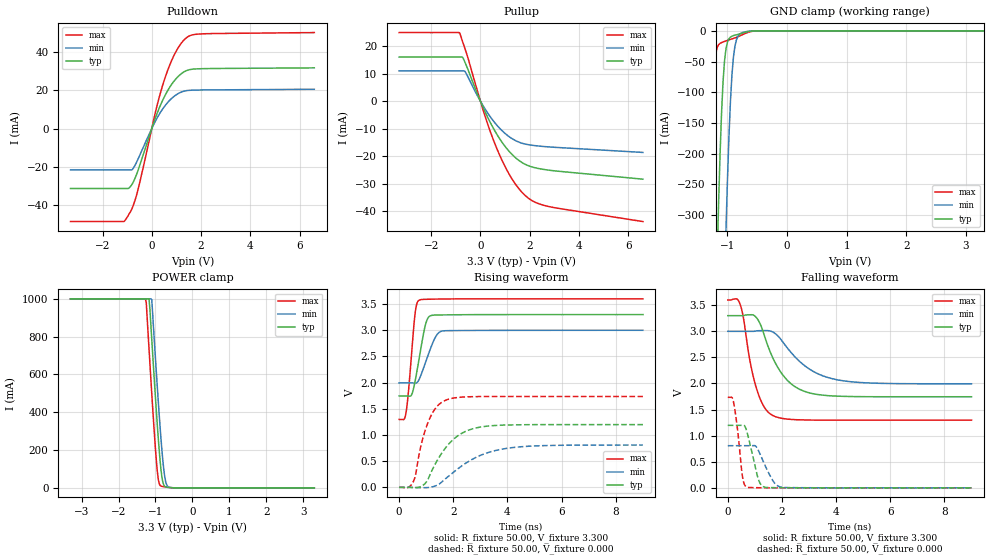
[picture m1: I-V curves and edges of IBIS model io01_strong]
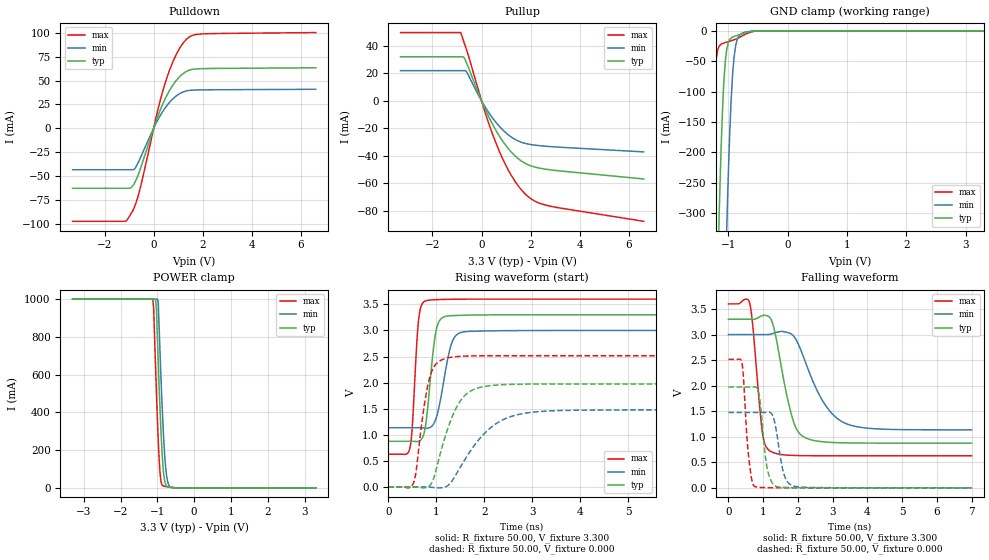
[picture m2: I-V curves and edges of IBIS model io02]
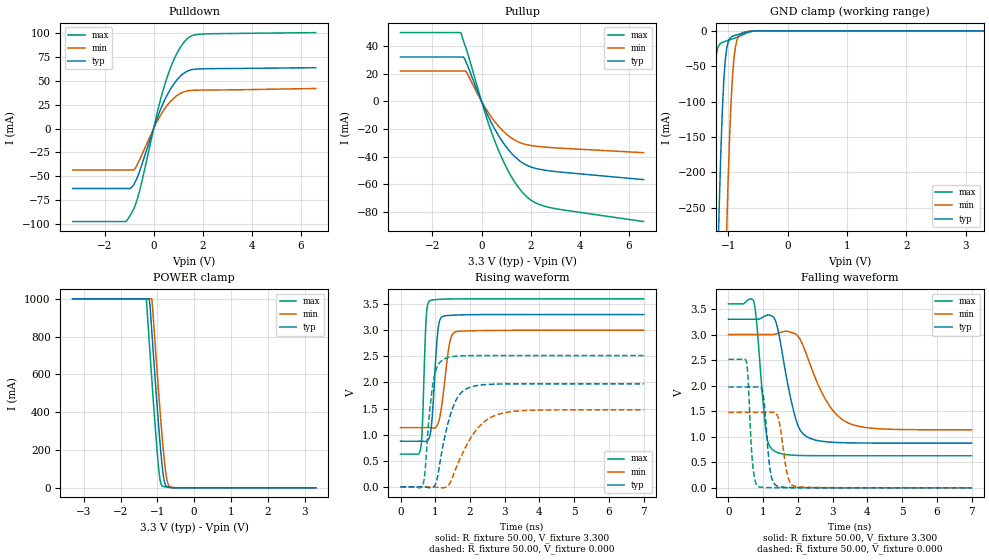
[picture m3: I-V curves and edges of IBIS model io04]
[IBIS Ver]   3.2
[File name]   rx630_177tflga.ibs
[File Rev]   2.00
[Date]   Sep 10, 2012
[Source]   From silicon level SPICE model at
   Renesas Electronics Corporation
[Notes]
|   Renesas Microcomputer RX630 Group
|   RX630 177pin TFLGA
|   VCCQ : 3.30V
|(1) This IBIS file checked the format with ibischk5.
|   Format Error and Warning are 0.
|(2) Temperature described Tj.
|   Tj[deg]
|   Typical   45.0
|   Minimum   105.0
|   Maximum   -40.0
|(3) History
|   Rev 1.00  2012.3.22
|   New creation by Hitachi ULSI Systems Co,.Ltd.
|   Rev 2.00  2012.09.10
|   Some IO Models were changed
|   by Renesas Electronics Corporation
[Disclaimer]
   This information is for modeling purposes only,
   and is not guaranteed.
[Copyright]   Copyright 2012, Renesas Electronics Corporation ,
   All Rights Reserved
[Component]   rx630_177tflga
[Manufacturer]  Renesas Electronics Corporation
[Package]
|   typ   min   max
R_pkg   358m   358m   358m
L_pkg   1.7nH   1.7nH   1.7nH
C_pkg   0.26pF   0.26pF   0.26pF
[Pin] signal_name   model_name
A1   AVSS0   GND
A2   AVCC0   POWER
A3   VREFL0   GND
A4   P42   io14
A5   P46   io14
A6   VCC   POWER
A7   VSS   GND
A8   P94   io07
A9   PK0   io04
A10   P97   io07
A11   PD6   io01
A12   P60   io07
A13   P63   io07
A14   PE1   io01
A15   PE2   io01
B1   P05   io02
B2   P07   io06
B3   P40   io14
B4   P41   io14
B5   P47   io14
B6   P91   io01
B7   P92   io01
B8   PD1   io01
B9   P96   io07
B10   PD4   io01
B11   PG1   io07
B12   PK3   io04
B13   P64   io07
B14   PE0   io01
B15   PE3   io01
C1   VREFL   GND
C2   VREFH   POWER
C3   VREFH0   POWER
C4   P43   io14
C5   P45   io14
C6   P90   io01
C7   PD0   io01
C8   PD2   io01
C9   PD3   io01
C10   PG0   io07
C11   PK2   io04
C12   P62   io07
C13   PE4   io01
C14   PK4   io04
C15   P70   io07
D1   P01   io01
D2   P02   io01
D3   P03   io02
D4   P00   io01
D5   P44   io14
D6   P93   io01
D7   P95   io07
D8   PK1   io04
D9   PD5   io01
D10   PD7   io01
D11   P61   io07
D12   PE5   io01
D13   PK5   io04
D14   PE7   io01
D15   P65   io07
E1   PJ5   io04
E2   EMLE   input06
E3   PF5   io04
E4   VSS   GND
E5   NC   NC
E12   PE6   io01
E13   PG2   io07
E14   PG3   io07
E15   P67   io08
F1   VBATT   POWER
F2   VCL   POWER
F3   PJ3   io04
F4   BSCANP   input03
F12   P66   io07
F13   PG4   io07
F14   PA0   io07
F15   VSS   GND
G1   XCIN   NC
G2   XCOUT   NC
G3   MD   io04
G4   PF4   io04
G12   PG5   io04
G13   PG6   io07
G14   PA1   io08
G15   VCC   POWER
H1   P37   io05
H2   VSS   GND
H3   RES#   input02
H4   P35   input01
H12   PA4   io08
H13   PA3   io08
H14   PA2   io08
H15   PG7   io07
J1   P36   io03
J2   VCC   POWER
J3   P34   io06
J4   PF3   io04
J12   PA5   io07
J13   PK6   io04
J14   PA7   io07
J15   PA6   io08
K1   P33   io06
K2   P32   io21
K3   PF2   io04
K4   PF1   io04
K12   PB2   io08
K13   P71   io07
K14   PK7   io04
K15   PB0   io08
L1   P31   io21
L2   P30   io21
L3   PF0   io04
L4   P25   io06
L12   PB6   io08
L13   PB3   io08
L14   PB1   io08
L15   P72   io07
M1   P27   io07
M2   P26   io07
M3   P24   io06
M4   P86   io04
M5   P13   io18
M6   P56   io08
M7   P54   io08
M8   P53   io04
M9   P50   io08
M10   PC5   io08
M11   P81   io06
M12   P77   io08
M13   PB7   io08
M14   PB5   io08
M15   PB4   io08
N1   PH5   io04
N2   P23   io06
N3   P22   io06
N4   P15   io06
N5   P12   io18
N6   P57   io08
N7   P55   io08
N8   PL2   io04
N9   P51   io08
N10   PC7   io08
N11   P82   io06
N12   PC3   io08
N13   PC0   io17
N14   P73   io07
N15   PL0   io04
P1   PH4   io04
P2   P17   io15
P3   P87   io04
P4   P14   io06
P5   P10   io04
P6   VCC_USB   POWER
P7   VSS_USB   GND
P8   PL3   io04
P9   P52   io08
P10   P83   io04
P11   PC6   io08
P12   PC4   io08
P13   PC2   io08
P14   P75   io08
P15   PL1   io04
R1   P21   io16
R2   P20   io16
R3   P16   io15
R4   P85   io04
R5   P11   io04
R6   USB0_DM   io09
R7   USB0_DP   io09
R8   PL4   io04
R9   P84   io04
R10   VSS   GND
R11   VCC   POWER
R12   P80   io06
R13   P76   io08
R14   P74   io08
R15   PC1   io17
[Diff Pin]   inv_pin   vdiff   tdelay_typ   tdelay_min   tdelay_max
R6   R7   0.000V   0.000s   NA   NA
[Model Selector]   io01
io01_strong   driver strength strong
io01_weak   driver strength weak
[Model Selector]   io07
io07_strong   driver strength strong
io07_weak   driver strength weak
[Model Selector]   io08
io08_strong   driver strength strong
io08_weak   driver strength weak
[Model Selector]   io15
io15a   driver strength strong
io15b   I2C buffer 1
[Model Selector]   io16
io16a   driver strength strong
io16b   I2C buffer 2
[Model Selector]   io17
io17a_strong   driver strength strong
io17a_weak   driver strength weak
io17b   I2C buffer 3
[Model Selector]   io18
io18a   driver strength strong
io18b   I2C buffer 4
| Models and submodels in the file (27): io01_strong (I/O), io01_weak (I/O), io02 (I/O), io03 (I/O), io04 (I/O), io05 (I/O), io06 (I/O), io07_strong (I/O), io07_weak (I/O), io08_strong (I/O), io08_weak (I/O), io09 (I/O), io14 (I/O), io15a (I/O), io15b (I/O_open_drain), io16a (I/O), io16b (I/O_open_drain), io17a_strong (I/O), io17a_weak (I/O), io17b (I/O_open_drain), io18a (I/O), io18b (I/O_open_drain), io21 (I/O), input01 (Input), input02 (Input), input03 (Input), input06 (Input)
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[Model]   io01_strong
Model_type   I/O
Polarity   Non-Inverting
Enable   Active-High
Vinl  =   0.660V
Vinh  =   2.640V
Vmeas =   1.650V
Cref  =   30.00pF
| variable   typ   min   max
C_comp   5.910pF   5.910pF   5.910pF
| variable   typ   min   max
[Temperature Range]   45.000   105.000   -40.000
| variable   typ   min   max
[Voltage Range]   3.300V   3.000V   3.600V
| variable   typ   min   max
[Pullup Reference]   3.300V   3.000V   3.600V
| variable   typ   min   max
[Pulldown Reference]   0.000V   0.000V   0.000V
| variable   typ   min   max
[POWER Clamp Reference] 3.300V   3.000V   3.600V
| variable   typ   min   max
[GND Clamp Reference]   0.000V   0.000V   0.000V
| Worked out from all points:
|   slope of the pulldown table from 0 to 0.495 V, typ, clamps not added: 30.7 ohm
|   slope of the pullup table from 0 to 0.495 V, typ, clamps not added: 52.9 ohm
|   GND clamp passes 1 mA (typ) near -0.63 V on its own axis
|   POWER clamp passes 1 mA (typ) near -0.58 V on its own axis
|   rising waveform, R_fixture 50.00, V_fixture 3.300: 20-80 % time 321ps typ, 432ps min, 222ps max; typ from 1.75 V to 3.3 V
|   rising waveform, R_fixture 50.00, V_fixture 0.000: 20-80 % time 961ps typ, 1.48ns min, 553ps max; typ from 0 V to 1.2 V
|   falling waveform, R_fixture 50.00, V_fixture 3.300: 20-80 % time 902ps typ, 1.27ns min, 542ps max; typ from 3.3 V to 1.75 V
|   falling waveform, R_fixture 50.00, V_fixture 0.000: 20-80 % time 324ps typ, 446ps min, 218ps max; typ from 1.2 V to 0 V
[Pulldown]
| io01_strong Pulldown rx630
| Thu Mar 22 17:15:49 2012
| voltage   I(typ)   I(min)   I(max)
-3.3V     -31.31mA   -21.63mA   -48.57mA
-1.15V    -31.31mA   -21.63mA   -48.57mA
-1.025V   -31.31mA   -21.63mA   -46.81mA
-800mV    -29.1mA    -21.49mA   -41.71mA
-600mV    -23.34mA   -17.13mA   -33.95mA
175mV     6.49mA     4.538mA    9.911mA
525mV     16.92mA    11.68mA    25.93mA
950mV     25.49mA    17.23mA    39.38mA
1.4V      30.18mA    19.75mA    47.31mA
1.7V      31.04mA    20.05mA    49.02mA
2.1V      31.26mA    20.14mA    49.45mA
6.6V      31.67mA    20.5mA     50.09mA
[Pullup]
| io01_strong Pullup rx630
| Thu Mar 22 17:15:49 2012
| voltage   I(typ)   I(min)   I(max)
-3.3V     16.04mA    10.98mA    24.94mA
-850mV    16.04mA    10.98mA    24.94mA
-725mV    15.94mA    10.98mA    21.66mA
-625mV    14.1mA     10.75mA    19.05mA
175mV     -3.59mA    -2.649mA   -5.083mA
700mV     -12.53mA   -9.072mA   -17.96mA
1V        -16.45mA   -11.75mA   -23.79mA
1.325V    -19.76mA   -13.87mA   -28.89mA
1.95V     -23.51mA   -15.85mA   -35.33mA
2.3V      -24.41mA   -16.28mA   -37.1mA
2.9V      -25.25mA   -16.74mA   -38.59mA
6.6V      -28.4mA    -18.67mA   -43.82mA
[GND Clamp]
| io01_strong GNDClamp rx630
| Thu Mar 22 17:15:49 2012
| voltage   I(typ)   I(min)   I(max)
-3.3V     -1A        -1A        -1A
-1.325V   -1A        -1A        -369.2mA
-1.3V     -928.6mA   -1A        -269.7mA
-1.25V    -694.8mA   -1A        -112.6mA
-1.175V   -376mA     -953.3mA   -27.44mA
-1.15V    -283.8mA   -837.7mA   -22.69mA
-1.075V   -83.42mA   -512.2mA   -18.16mA
-1.025V   -28.94mA   -323mA     -16.39mA
-925mV    -8.707mA   -71.38mA   -13.1mA
-850mV    -6.468mA   -14.65mA   -10.64mA
-675mV    -1.81mA    -1.082mA   -3.186mA
3.3V      0A         0A         0A
[POWER Clamp]
| io01_strong PWRClamp rx630
| Thu Mar 22 17:15:49 2012
| voltage   I(typ)   I(min)   I(max)
-3.3V     1A         1A         1A
-1.275V   1A         1A         1A
-1.25V    1A         1A         982.1mA
-1.175V   1A         1A         736.6mA
-1.1V     784.3mA    995.9mA    498mA
-1V       476.2mA    683.1mA    204.7mA
-950mV    332.1mA    533mA      87.52mA
-875mV    143.3mA    321.7mA    12.76mA
-825mV    55.42mA    197.2mA    7.873mA
-750mV    8.12mA     59.94mA    5.513mA
-625mV    1.619mA    2.607mA    2.132mA
3.3V      0A         0A         0A
[Ramp]
dV/dt_r   0.719/960.74p  0.485/1.48n   1.041/552.35p
dV/dt_f   0.933/901.13p  0.604/1.27n   1.382/541.71p
R_load = 50.00ohm
[Rising Waveform]
| io01_strong Rising-High rx630
| Thu Mar 22 17:15:49 2012
R_fixture = 50.00
V_fixture = 3.300
V_fixture_min = 3.000
V_fixture_max = 3.600
C_fixture = 0.00pF
| Time   V(typ)   V(min)   V(max)
0s        1.746V     1.994V     1.297V
250ps     1.746V     1.994V     1.413V
450ps     1.759V     1.994V     2.489V
580ps     2.004V     1.989V     3.28V
645ps     2.183V     1.996V     3.491V
740ps     2.465V     2.064V     3.575V
1.045ns   3.216V     2.49V      3.592V
1.35ns    3.291V     2.878V     3.596V
1.585ns   3.293V     2.985V     3.598V
9ns       3.3V       3V         3.6V
[Rising Waveform]
| io01_strong Rising-Low rx630
| Thu Mar 22 17:15:49 2012
R_fixture = 50.00
V_fixture = 0.000
C_fixture = 0.00pF
| Time   V(typ)   V(min)   V(max)
0s        0V         0V         0V
510ps     -7mV       0V         95mV
605ps     -9mV       -1mV       236mV
840ps     25mV       -7mV       868mV
1.075ns   164mV      -4mV       1.25V
1.385ns   494mV      37mV       1.537V
1.755ns   781mV      183mV      1.672V
2.55ns    1.09V      490mV      1.729V
3.975ns   1.191V     745mV      1.735V
9ns       1.198V     808mV      1.735V
[Falling Waveform]
| io01_strong Falling-High rx630
| Thu Mar 22 17:15:49 2012
R_fixture = 50.00
V_fixture = 3.300
V_fixture_min = 3.000
V_fixture_max = 3.600
C_fixture = 0.00pF
| Time   V(typ)   V(min)   V(max)
0s        3.3V       3V         3.6V
445ps     3.3V       3V         3.533V
575ps     3.301V     3V         3.268V
825ps     3.317V     3V         2.418V
1.03ns    3.279V     3.006V     1.959V
1.325ns   2.961V     3.013V     1.567V
1.65ns    2.506V     2.99V      1.39V
2.46ns    1.947V     2.523V     1.308V
3.835ns   1.763V     2.095V     1.297V
9ns       1.746V     1.994V     1.297V
[Falling Waveform]
| io01_strong Falling-Low rx630
| Thu Mar 22 17:15:49 2012
R_fixture = 50.00
V_fixture = 0.000
C_fixture = 0.00pF
| Time   V(typ)   V(min)   V(max)
0s        1.198V     808mV      1.735V
210ps     1.198V     808mV      1.65V
350ps     1.198V     808mV      1.163V
545ps     1.199V     808mV      210mV
710ps     1.068V     808mV      13mV
1.12ns    182mV      727mV      3mV
1.35ns    15mV       460mV      1mV
1.71ns    4mV        104mV      1mV
2.015ns   2mV        10mV       0V
9ns       0V         0V         0V
[Model]   io02
Model_type   I/O
Polarity   Non-Inverting
Enable   Active-High
Vinl  =   0.660V
Vinh  =   2.640V
Vmeas =   1.650V
Cref  =   30.00pF
| variable   typ   min   max
C_comp   4.810pF   4.810pF   4.810pF
| variable   typ   min   max
[Temperature Range]   45.000   105.000   -40.000
| variable   typ   min   max
[Voltage Range]   3.300V   3.000V   3.600V
| variable   typ   min   max
[Pullup Reference]   3.300V   3.000V   3.600V
| variable   typ   min   max
[Pulldown Reference]   0.000V   0.000V   0.000V
| variable   typ   min   max
[POWER Clamp Reference] 3.300V   3.000V   3.600V
| variable   typ   min   max
[GND Clamp Reference]   0.000V   0.000V   0.000V
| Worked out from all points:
|   slope of the pulldown table from 0 to 0.495 V, typ, clamps not added: 15.3 ohm
|   slope of the pullup table from 0 to 0.495 V, typ, clamps not added: 26.5 ohm
|   GND clamp passes 1 mA (typ) near -0.60 V on its own axis
|   POWER clamp passes 1 mA (typ) near -0.56 V on its own axis
|   rising waveform, R_fixture 50.00, V_fixture 3.300: 20-80 % time 160ps typ, 229ps min, 107ps max; typ from 0.875 V to 3.3 V
|   rising waveform, R_fixture 50.00, V_fixture 0.000: 20-80 % time 439ps typ, 750ps min, 233ps max; typ from 0 V to 1.97 V
|   falling waveform, R_fixture 50.00, V_fixture 3.300: 20-80 % time 438ps typ, 788ps min, 230ps max; typ from 3.3 V to 0.875 V
|   falling waveform, R_fixture 50.00, V_fixture 0.000: 20-80 % time 184ps typ, 224ps min, 154ps max; typ from 1.97 V to 0 V
[Pulldown]
| io02_strong Pulldown rx630
| Thu Mar 22 17:15:49 2012
| voltage   I(typ)   I(min)   I(max)
-3.3V     -62.65mA   -43.27mA   -97.17mA
-1.15V    -62.65mA   -43.27mA   -97.17mA
-1.025V   -62.65mA   -43.27mA   -93.54mA
-800mV    -58.14mA   -42.96mA   -83.35mA
-600mV    -46.61mA   -34.21mA   -67.78mA
175mV     12.96mA    9.063mA    19.79mA
550mV     35.03mA    24.16mA    53.7mA
950mV     50.92mA    34.42mA    78.67mA
1.4V      60.32mA    39.47mA    94.54mA
1.7V      62.04mA    40.07mA    97.97mA
2.1V      62.48mA    40.25mA    98.84mA
6.6V      63.3mA     40.84mA    100.1mA
[Pullup]
| io02_strong Pullup rx630
| Thu Mar 22 17:15:49 2012
| voltage   I(typ)   I(min)   I(max)
-3.3V     32.07mA    21.98mA    49.71mA
-850mV    32.07mA    21.98mA    49.71mA
-725mV    31.79mA    21.98mA    43.1mA
-625mV    28.07mA    21.44mA    37.9mA
150mV     -6.167mA   -4.559mA   -8.713mA
675mV     -24.26mA   -17.6mA    -34.7mA
975mV     -32.23mA   -23.07mA   -46.52mA
1.3V      -39mA      -27.43mA   -56.92mA
1.925V    -46.81mA   -31.61mA   -70.21mA
2.3V      -48.81mA   -32.55mA   -74.14mA
2.8V      -50.28mA   -33.35mA   -76.77mA
6.6V      -56.92mA   -37.21mA   -87.76mA
[GND Clamp]
| io02_strong GNDClamp rx630
| Thu Mar 22 17:15:49 2012
| voltage   I(typ)   I(min)   I(max)
-3.3V     -1A        -1A        -1A
-1.325V   -1A        -1A        -406.6mA
-1.3V     -983.2mA   -1A        -299.4mA
-1.225V   -615mA     -1A        -75.45mA
-1.175V   -395.1mA   -992.5mA   -30.98mA
-1.15V    -297.6mA   -869.7mA   -25.1mA
-1.075V   -87.49mA   -526mA     -20.19mA
-1.025V   -30.91mA   -328.2mA   -18.56mA
-925mV    -10.2mA    -71.04mA   -15.59mA
-850mV    -7.712mA   -14.99mA   -12.74mA
-675mV    -2.503mA   -1.438mA   -4.223mA
3.3V      0A         0A         0A
[POWER Clamp]
| io02_strong PWRClamp rx630
| Thu Mar 22 17:15:49 2012
| voltage   I(typ)   I(min)   I(max)
-3.3V     1A         1A         1A
-1.125V   1A         1A         1A
-1.1V     1A         1A         952.1mA
-1.05V    1A         1A         650.2mA
-1.025V   951.6mA    1A         507.1mA
-975mV    665.2mA    983.6mA    250.2mA
-925mV    406mA      705.8mA    73.52mA
-850mV    120.7mA    345.8mA    11.13mA
-800mV    34.79mA    171.7mA    8.224mA
-750mV    9.544mA    66.61mA    6.556mA
-625mV    2.042mA    3.124mA    2.737mA
3.3V      0A         0A         0A
[Ramp]
dV/dt_r   1.184/438.21p  0.886/749.00p  1.509/232.71p
dV/dt_f   1.455/438.02p  1.119/787.01p  1.783/229.46p
R_load = 50.00ohm
[Rising Waveform]
| io02_strong Rising-High rx630
| Thu Mar 22 17:15:49 2012
R_fixture = 50.00
V_fixture = 3.300
V_fixture_min = 3.000
V_fixture_max = 3.600
C_fixture = 0.00pF
| Time   V(typ)   V(min)   V(max)
0s        875mV      1.135V     628mV
445ps     876mV      1.135V     734mV
495ps     875mV      1.135V     1.111V
625ps     873mV      1.135V     3.163V
760ps     1.097V     1.13V      3.561V
975ps     2.901V     1.27V      3.589V
1.16ns    3.261V     2.067V     3.595V
1.345ns   3.284V     2.816V     3.598V
1.575ns   3.291V     2.973V     3.599V
7ns       3.3V       3V         3.6V
[Rising Waveform]
| io02_strong Rising-Low rx630
| Thu Mar 22 17:15:49 2012
R_fixture = 50.00
V_fixture = 0.000
C_fixture = 0.00pF
| Time   V(typ)   V(min)   V(max)
0s        0V         0V         0V
520ps     0V         0V         67mV
840ps     9mV        -4mV       2.022V
965ps     227mV      -13mV      2.324V
1.155ns   880mV      -9mV       2.452V
1.39ns    1.472V     210mV      2.496V
1.65ns    1.799V     608mV      2.51V
2.09ns    1.938V     1.104V     2.515V
2.6ns     1.967V     1.363V     2.515V
7ns       1.974V     1.476V     2.515V
[Falling Waveform]
| io02_strong Falling-High rx630
| Thu Mar 22 17:15:49 2012
R_fixture = 50.00
V_fixture = 3.300
V_fixture_min = 3.000
V_fixture_max = 3.600
C_fixture = 0.00pF
| Time   V(typ)   V(min)   V(max)
0s        3.3V       3V         3.6V
610ps     3.3V       3V         3.618V
700ps     3.299V     3V         3.177V
985ps     3.373V     3V         1.049V
1.205ns   3.323V     3.007V     719mV
1.815ns   1.429V     3.009V     637mV
2.145ns   1.007V     2.591V     631mV
2.74ns    900mV      1.672V     629mV
3.33ns    881mV      1.274V     628mV
7ns       875mV      1.135V     628mV
[Falling Waveform]
| io02_strong Falling-Low rx630
| Thu Mar 22 17:15:49 2012
R_fixture = 50.00
V_fixture = 0.000
C_fixture = 0.00pF
| Time   V(typ)   V(min)   V(max)
0s        1.974V     1.476V     2.515V
385ps     1.974V     1.476V     2.454V
570ps     1.974V     1.476V     683mV
755ps     1.978V     1.476V     29mV
890ps     1.793V     1.476V     10mV
1.125ns   352mV      1.48V      4mV
1.36ns    32mV       1.19V      2mV
1.61ns    9mV        242mV      1mV
1.88ns    4mV        36mV       0V
7ns       0V         0V         0V
[Model]   io04
Model_type   I/O
Polarity   Non-Inverting
Enable   Active-High
Vinl  =   0.660V
Vinh  =   2.640V
Vmeas =   1.650V
Cref  =   30.00pF
| variable   typ   min   max
C_comp   4.420pF   4.420pF   4.420pF
| variable   typ   min   max
[Temperature Range]   45.000   105.000   -40.000
| variable   typ   min   max
[Voltage Range]   3.300V   3.000V   3.600V
| variable   typ   min   max
[Pullup Reference]   3.300V   3.000V   3.600V
| variable   typ   min   max
[Pulldown Reference]   0.000V   0.000V   0.000V
| variable   typ   min   max
[POWER Clamp Reference] 3.300V   3.000V   3.600V
| variable   typ   min   max
[GND Clamp Reference]   0.000V   0.000V   0.000V
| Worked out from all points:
|   slope of the pulldown table from 0 to 0.495 V, typ, clamps not added: 15.4 ohm
|   slope of the pullup table from 0 to 0.495 V, typ, clamps not added: 26.5 ohm
|   GND clamp passes 1 mA (typ) near -0.64 V on its own axis
|   POWER clamp passes 1 mA (typ) near -0.59 V on its own axis
|   rising waveform, R_fixture 50.00, V_fixture 3.300: 20-80 % time 137ps typ, 205ps min, 88.9ps max; typ from 0.875 V to 3.3 V
|   rising waveform, R_fixture 50.00, V_fixture 0.000: 20-80 % time 423ps typ, 741ps min, 213ps max; typ from 0 V to 1.97 V
|   falling waveform, R_fixture 50.00, V_fixture 3.300: 20-80 % time 429ps typ, 779ps min, 219ps max; typ from 3.3 V to 0.875 V
|   falling waveform, R_fixture 50.00, V_fixture 0.000: 20-80 % time 149ps typ, 194ps min, 116ps max; typ from 1.97 V to 0 V
[Pulldown]
| io04_strong Pulldown rx630
| Thu Mar 22 17:15:49 2012
| voltage   I(typ)   I(min)   I(max)
-3.3V     -62.62mA   -43.25mA   -97.14mA
-1.15V    -62.62mA   -43.25mA   -97.14mA
-1.025V   -62.62mA   -43.25mA   -93.52mA
-800mV    -58.13mA   -42.94mA   -83.32mA
-600mV    -46.6mA    -34.2mA    -67.76mA
175mV     12.96mA    9.062mA    19.78mA
550mV     35.03mA    24.16mA    53.68mA
950mV     50.91mA    34.42mA    78.65mA
1.4V      60.32mA    39.47mA    94.53mA
1.7V      62.04mA    40.07mA    97.97mA
2.1V      62.47mA    40.25mA    98.84mA
6.6V      63.56mA    41.89mA    100.3mA
[Pullup]
| io04_strong Pullup rx630
| Thu Mar 22 17:15:49 2012
| voltage   I(typ)   I(min)   I(max)
-3.3V     32.04mA    21.95mA    49.68mA
-850mV    32.04mA    21.95mA    49.68mA
-725mV    31.77mA    21.95mA    43.08mA
-625mV    28.06mA    21.43mA    37.88mA
150mV     -6.165mA   -4.558mA   -8.71mA
675mV     -24.25mA   -17.59mA   -34.7mA
1V        -32.82mA   -23.46mA   -47.4mA
1.3V      -39mA      -27.43mA   -56.91mA
1.925V    -46.81mA   -31.61mA   -70.21mA
2.3V      -48.81mA   -32.55mA   -74.14mA
2.9V      -50.5mA    -33.47mA   -77.15mA
6.6V      -56.53mA   -37.08mA   -86.83mA
[GND Clamp]
| io04_strong GNDClamp rx630
| Thu Mar 22 17:15:49 2012
| voltage   I(typ)   I(min)   I(max)
-3.3V     -1A        -1A        -1A
-1.325V   -916.4mA   -1A        -321.6mA
-1.225V   -508.3mA   -1A        -56.05mA
-1.175V   -327.1mA   -831.8mA   -23.6mA
-1.15V    -246.5mA   -730.6mA   -19.51mA
-1.075V   -71.99mA   -445.9mA   -15.62mA
-1.025V   -24.89mA   -280.5mA   -14.09mA
-975mV    -11.12mA   -147.9mA   -12.65mA
-925mV    -7.484mA   -61.53mA   -11.26mA
-850mV    -5.559mA   -12.59mA   -9.146mA
-675mV    -1.555mA   -930uA     -2.738mA
3.3V      0A         0A         0A
[POWER Clamp]
| io04_strong PWRClamp rx630
| Thu Mar 22 17:15:49 2012
| voltage   I(typ)   I(min)   I(max)
-3.3V     1A         1A         1A
-1.3V     1A         1A         1A
-1.225V   1A         1A         787.8mA
-1.2V     968.8mA    1A         716.2mA
-1.15V    827mA      1A         574.7mA
-975mV    353.5mA    532.6mA    124.6mA
-925mV    232.2mA    403.9mA    41.33mA
-875mV    126.2mA    282.6mA    11.35mA
-825mV    48.99mA    173.5mA    7.014mA
-750mV    7.221mA    53mA       4.912mA
-625mV    1.442mA    2.321mA    1.9mA
3.3V      0A         0A         0A
[Ramp]
dV/dt_r   1.184/423.57p  0.886/740.07p  1.509/212.85p
dV/dt_f   1.455/428.81p  1.119/778.62p  1.783/218.73p
R_load = 50.00ohm
[Rising Waveform]
| io04_strong Rising-High rx630
| Thu Mar 22 17:15:49 2012
R_fixture = 50.00
V_fixture = 3.300
V_fixture_min = 3.000
V_fixture_max = 3.600
C_fixture = 0.00pF
| Time   V(typ)   V(min)   V(max)
0s        875mV      1.135V     628mV
575ps     876mV      1.135V     720mV
625ps     875mV      1.135V     1.101V
740ps     871mV      1.136V     3.247V
840ps     969mV      1.134V     3.562V
1.075ns   2.982V     1.207V     3.588V
1.205ns   3.261V     1.649V     3.593V
1.4ns     3.283V     2.704V     3.597V
1.57ns    3.289V     2.964V     3.599V
7ns       3.3V       3V         3.6V
[Rising Waveform]
| io04_strong Rising-Low rx630
| Thu Mar 22 17:15:49 2012
R_fixture = 50.00
V_fixture = 0.000
C_fixture = 0.00pF
| Time   V(typ)   V(min)   V(max)
0s        0V         0V         0V
655ps     0V         0V         70mV
835ps     -17mV      0V         1.423V
945ps     1mV        -2mV       2.018V
1.06ns    173mV      -9mV       2.308V
1.245ns   869mV      -16mV      2.444V
1.705ns   1.772V     526mV      2.508V
2.195ns   1.94V      1.102V     2.514V
2.685ns   1.967V     1.358V     2.515V
7ns       1.973V     1.476V     2.515V
[Falling Waveform]
| io04_strong Falling-High rx630
| Thu Mar 22 17:15:49 2012
R_fixture = 50.00
V_fixture = 3.300
V_fixture_min = 3.000
V_fixture_max = 3.600
C_fixture = 0.00pF
| Time   V(typ)   V(min)   V(max)
0s        3.3V       3V         3.6V
730ps     3.3V       3V         3.645V
810ps     3.299V     3V         3.25V
1.09ns    3.374V     3V         1.055V
1.325ns   3.313V     3.004V     720mV
1.91ns    1.416V     3.019V     637mV
2.245ns   1.005V     2.613V     631mV
2.85ns    899mV      1.667V     629mV
3.43ns    881mV      1.275V     628mV
7ns       875mV      1.135V     628mV
[Falling Waveform]
| io04_strong Falling-Low rx630
| Thu Mar 22 17:15:49 2012
R_fixture = 50.00
V_fixture = 0.000
C_fixture = 0.00pF
| Time   V(typ)   V(min)   V(max)
0s        1.973V     1.476V     2.515V
515ps     1.973V     1.476V     2.467V
695ps     1.973V     1.476V     474mV
845ps     1.975V     1.476V     28mV
1ns       1.82V      1.476V     10mV
1.225ns   253mV      1.478V     4mV
1.415ns   31mV       1.405V     2mV
1.69ns    9mV        278mV      1mV
1.9ns     5mV        31mV       0V
7ns       0V         0V         0V
